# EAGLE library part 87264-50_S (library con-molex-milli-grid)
RECEPTACAL
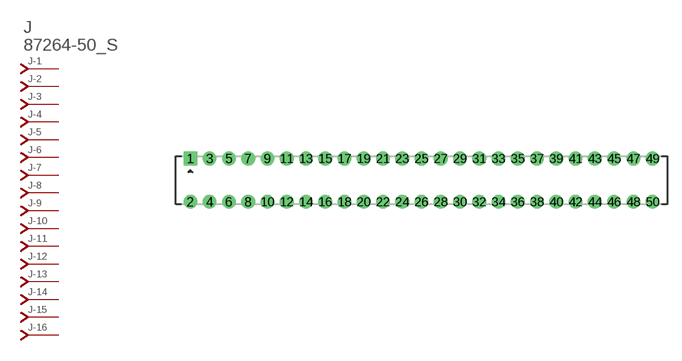
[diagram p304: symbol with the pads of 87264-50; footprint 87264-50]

Designator prefix J; gates -1=J-NV -2=J-N -3=J-N -4=J-N -5=J-N -6=J-N -7=J-N -8=J-N -9=J-N -10=J-N -11=J-N -12=J-N -13=J-N -14=J-N -15=J-N -16=J-N -17=J-N -18=J-N -19=J-N -20=J-N -21=J-N -22=J-N -23=J-N -24=J-N -25=J-N -26=J-N -27=J-N -28=J-N -29=J-N -30=J-N -31=J-N -32=J-N -33=J-N -34=J-N -35=J-N -36=J-N -37=J-N -38=J-N -39=J-N -40=J-N -41=J-N -42=J-N -43=J-N -44=J-N -45=J-N -46=J-N -47=J-N -48=J-N -49=J-N -50=J-N

## 87264-50_S  [87264-50]
1  -1:J  pas
2  -2:J  pas
3  -3:J  pas
4  -4:J  pas
5  -5:J  pas
6  -6:J  pas
7  -7:J  pas
8  -8:J  pas
9  -9:J  pas
10  -10:J  pas
11  -11:J  pas
12  -12:J  pas
13  -13:J  pas
14  -14:J  pas
15  -15:J  pas
16  -16:J  pas
17  -17:J  pas
18  -18:J  pas
19  -19:J  pas
20  -20:J  pas
21  -21:J  pas
22  -22:J  pas
23  -23:J  pas
24  -24:J  pas
25  -25:J  pas
26  -26:J  pas
27  -27:J  pas
28  -28:J  pas
29  -29:J  pas
30  -30:J  pas
31  -31:J  pas
32  -32:J  pas
33  -33:J  pas
34  -34:J  pas
35  -35:J  pas
36  -36:J  pas
37  -37:J  pas
38  -38:J  pas
39  -39:J  pas
40  -40:J  pas
41  -41:J  pas
42  -42:J  pas
43  -43:J  pas
44  -44:J  pas
45  -45:J  pas
46  -46:J  pas
47  -47:J  pas
48  -48:J  pas
49  -49:J  pas
50  -50:J  pas

## Footprint 87264-50 (pad centres in mm)
RECEPTACAL Dual Row, Side Entry
drill 0.914 square: 1 -24,2.25
drill 0.914: 2 -24,-2.25; 3 -22,2.25; 4 -22,-2.25; 5 -20,2.25; 6 -20,-2.25; 7 -18,2.25; 8 -18,-2.25; 9 -16,2.25; 10 -16,-2.25; 11 -14,2.25; 12 -14,-2.25; 13 -12,2.25; 14 -12,-2.25; 15 -10,2.25; 16 -10,-2.25; 17 -8,2.25; 18 -8,-2.25; 19 -6,2.25; 20 -6,-2.25; 21 -4,2.25; 22 -4,-2.25; 23 -2,2.25; 24 -2,-2.25; 25 0,2.25; 26 0,-2.25; 27 2,2.25; 28 2,-2.25; 29 4,2.25; 30 4,-2.25; 31 6,2.25; 32 6,-2.25; 33 8,2.25; 34 8,-2.25; 35 10,2.25; 36 10,-2.25; 37 12,2.25; 38 12,-2.25; 39 14,2.25; 40 14,-2.25; 41 16,2.25; 42 16,-2.25; 43 18,2.25; 44 18,-2.25; 45 20,2.25; 46 20,-2.25; 47 22,2.25; 48 22,-2.25; 49 24,2.25; 50 24,-2.25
